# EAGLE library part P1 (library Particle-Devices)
Particle P1 module (WiFi with antenna) Product datasheet: here Github : Particle devices library
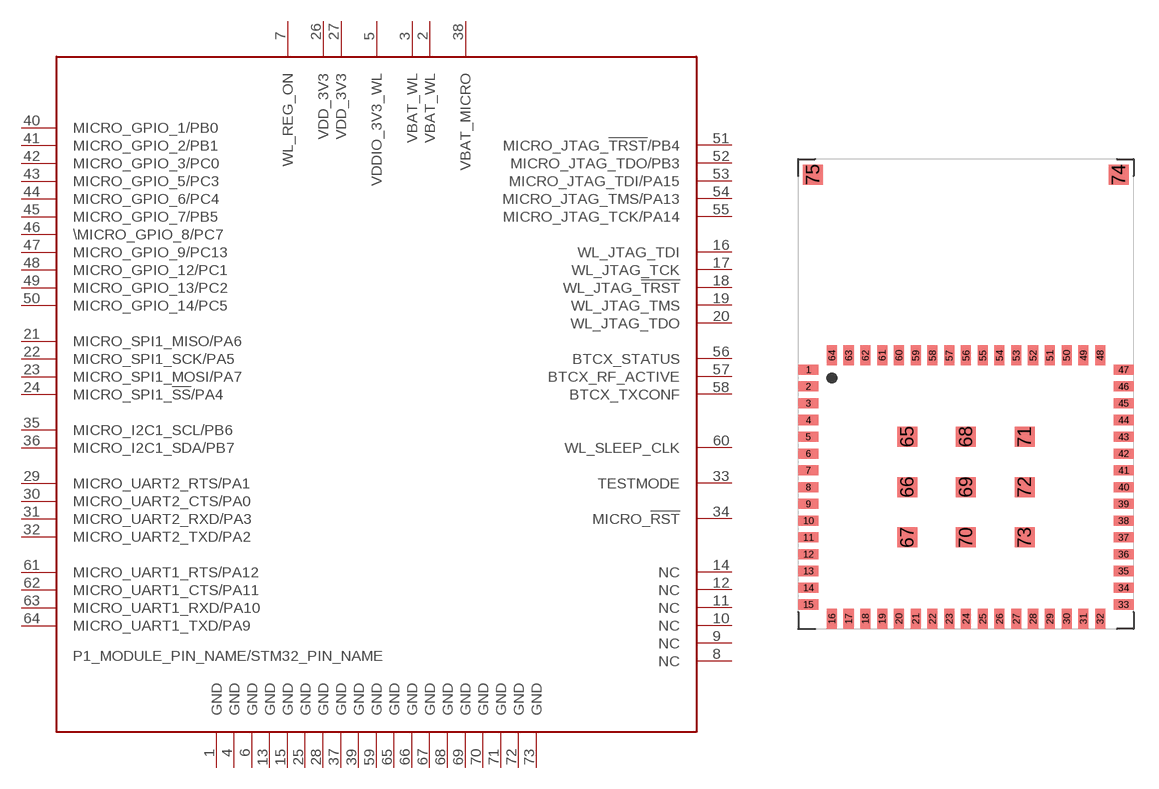
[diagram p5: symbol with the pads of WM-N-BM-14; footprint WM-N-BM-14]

Designator prefix -

## P1  [WM-N-BM-14]
1  GND
2  VBAT_WL
3  VBAT_WL
4  GND
5  VDDIO_3V3_WL
6  GND
7  WL_REG_ON
8  NC
9  NC
10  NC
11  NC
12  NC
13  GND
14  NC
15  GND
16  WL_JTAG_TDI
17  WL_JTAG_TCK
18  WL_JTAG_!TRST!
19  WL_JTAG_TMS
20  WL_JTAG_TDO
21  MICRO_SPI1_MISO/PA6
22  MICRO_SPI1_SCK/PA5
23  MICRO_SPI1_MOSI/PA7
24  MICRO_SPI1_!SS!/PA4
25  GND
26  VDD_3V3
27  VDD_3V3
28  GND
29  MICRO_UART2_RTS/PA1
30  MICRO_UART2_CTS/PA0
31  MICRO_UART2_RXD/PA3
32  MICRO_UART2_TXD/PA2
33  TESTMODE
34  MICRO_!RST!
35  MICRO_I2C1_SCL/PB6
36  MICRO_I2C1_SDA/PB7
37  GND
38  VBAT_MICRO
39  GND
40  MICRO_GPIO_1/PB0
41  MICRO_GPIO_2/PB1
42  MICRO_GPIO_3/PC0
43  MICRO_GPIO_5/PC3
44  MICRO_GPIO_6/PC4
45  MICRO_GPIO_7/PB5
46  \MICRO_GPIO_8/PC7
47  MICRO_GPIO_9/PC13
48  MICRO_GPIO_12/PC1
49  MICRO_GPIO_13/PC2
50  MICRO_GPIO_14/PC5
51  MICRO_JTAG_!TRST!/PB4
52  MICRO_JTAG_TDO/PB3
53  MICRO_JTAG_TDI/PA15
54  MICRO_JTAG_TMS/PA13
55  MICRO_JTAG_TCK/PA14
56  BTCX_STATUS
57  BTCX_RF_ACTIVE
58  BTCX_TXCONF
59  GND
60  WL_SLEEP_CLK
61  MICRO_UART1_RTS/PA12
62  MICRO_UART1_CTS/PA11
63  MICRO_UART1_RXD/PA10
64  MICRO_UART1_TXD/PA9
65  GND
66  GND
67  GND
68  GND
69  GND
70  GND
71  GND
72  GND
73  GND

## Footprint WM-N-BM-14 (pad centres in mm)
smd 1.2 x 0.6: 1 0.6,15.45; 2 0.6,14.45; 3 0.6,13.45; 4 0.6,12.45; 5 0.6,11.45; 6 0.6,10.45; 7 0.6,9.45; 8 0.6,8.45; 9 0.6,7.45; 10 0.6,6.45; 11 0.6,5.45; 12 0.6,4.45; 13 0.6,3.45; 14 0.6,2.45; 15 0.6,1.45; 33 19.4,1.45; 34 19.4,2.45; 35 19.4,3.45; 36 19.4,4.45; 37 19.4,5.45; 38 19.4,6.45; 39 19.4,7.45; 40 19.4,8.45; 41 19.4,9.45; 42 19.4,10.45; 43 19.4,11.45; 44 19.4,12.45; 45 19.4,13.45; 46 19.4,14.45; 47 19.4,15.45
smd 0.6 x 1.2: 16 2,0.6; 17 3,0.6; 18 4,0.6; 19 5,0.6; 20 6,0.6; 21 7,0.6; 22 8,0.6; 23 9,0.6; 24 10,0.6; 25 11,0.6; 26 12,0.6; 27 13,0.6; 28 14,0.6; 29 15,0.6; 30 16,0.6; 31 17,0.6; 32 18,0.6; 48 18,16.3; 49 17,16.3; 50 16,16.3; 51 15,16.3; 52 14,16.3; 53 13,16.3; 54 12,16.3; 55 11,16.3; 56 10,16.3; 57 9,16.3; 58 8,16.3; 59 7,16.3; 60 6,16.3; 61 5,16.3; 62 4,16.3; 63 3,16.3; 64 2,16.3
smd 1.2 x 1.2: 65 6.5,11.45; 66 6.5,8.45; 67 6.5,5.45; 68 10,11.45; 69 10,8.45; 70 10,5.45; 71 13.5,11.45; 72 13.5,8.45; 73 13.5,5.45; 74 19.12,27.07; 75 0.88,27.07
